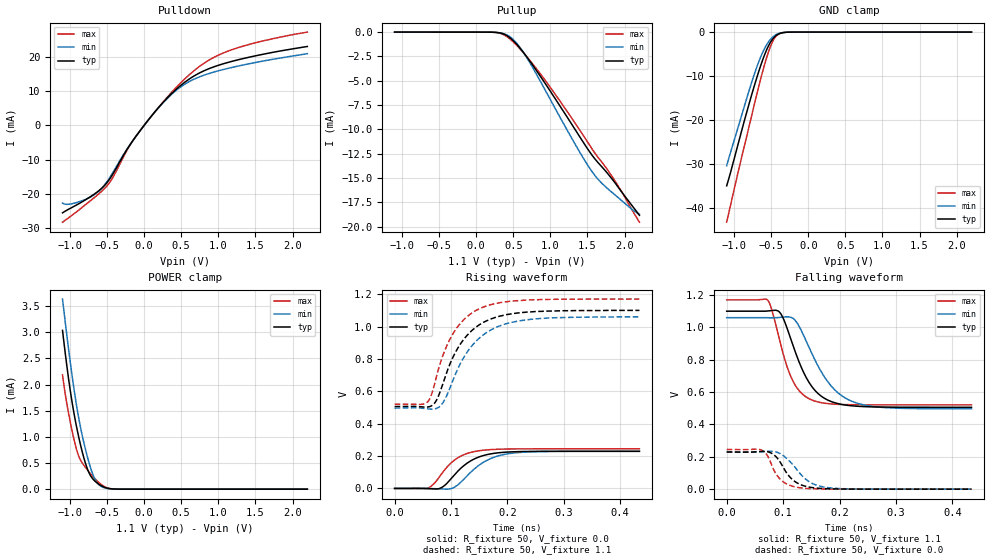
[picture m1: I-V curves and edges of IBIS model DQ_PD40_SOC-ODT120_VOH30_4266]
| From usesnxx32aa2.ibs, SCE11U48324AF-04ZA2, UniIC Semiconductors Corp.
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| DQ_PD40_SOC-ODT120_VOH30_4266
| (40 Ohm Pulldown, 120 Ohm System ODT Setting, VOH=VDDQ/3.0, 3200-4266Mbps)
[Model]   DQ_PD40_SOC-ODT120_VOH30_4266
Model_type   I/O
Vinl = 123.333mV
Vinh = 243.333mV
Vmeas = 183.333mV
Vref = 0.0mV
Cref = 0.0pF
Rref = 120.000Ohm
|   typ   min   max
|C_comp   0.797pF   0.747pF   0.847pF
C_comp_pullup   0.3985pF   0.3735pF   0.4235pF
C_comp_pulldown   0.3985pF   0.3735pF   0.4235pF
| Note: C_comp changes when the ODT circuit is enabled.
[Model Spec]
| Input threshold voltage corners
Vinl   0.1233V   0.1167V   0.1350V
Vinh   0.2433V   0.2367V   0.2550V
| Measurement voltage corners
Vmeas   0.1833V   0.1767V   0.1950V
| Timing spec test load voltage corners
Vref   0.0000V   0.0000V   0.0000V
| Dynamic Overshoot Parameters from LPDDR4 Specification
D_overshoot_ampl_h   0.30   NA   NA
D_overshoot_ampl_l   0.30   NA   NA
D_overshoot_area_h   0.1n   NA   NA
D_overshoot_area_l   0.1n   NA   NA
[Receiver Thresholds]
Vth   = 0.1833V
Vth_min  = 0.1800V
Vth_max  = 0.1866V
Vinh_ac  = 0.060V
Vinh_dc  = 0.060V
Vinl_ac  = -0.060V
Vinl_dc  = -0.060V
Tslew_ac = 5.000ns |Not specified, so set to high value
Threshold_sensitivity = 0.1667
Reference_supply Pullup_ref
[Voltage Range]   1.1000V   1.0600V   1.1700V
[Pullup Reference]   1.1000V   1.0600V   1.1700V
| Junction Temperature (Ambient temp is 35C typ 95C min -40C max)
[Temperature Range]   50.0   110.0   -40.0
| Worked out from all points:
|   slope of the pulldown table from 0 to 0.165 V, typ, clamps not added: 37 ohm
|   slope of the pullup table from 0 to 0.165 V, typ, clamps not added: 39.2 kohm
|   GND clamp passes 1 mA (typ) near -0.45 V on its own axis
|   POWER clamp passes 1 mA (typ) near -0.88 V on its own axis
|   rising waveform, R_fixture 50, V_fixture 0.0: 20-80 % time 45.7ps typ, 49.8ps min, 40.7ps max; typ from 0 V to 0.23 V
|   falling waveform, R_fixture 50, V_fixture 1.1: 20-80 % time 44.6ps typ, 56.1ps min, 34.9ps max; typ from 1.1 V to 0.506 V
|   rising waveform, R_fixture 50, V_fixture 1.1: 20-80 % time 55.4ps typ, 59.8ps min, 50.8ps max; typ from 0.506 V to 1.1 V
|   falling waveform, R_fixture 50, V_fixture 0.0: 20-80 % time 29.8ps typ, 37.9ps min, 24.9ps max; typ from 0.23 V to 0 V
[Pulldown]
|   Voltage   I(typ)   I(min)   I(max)
-1.1V     -25.52mA   -22.67mA   -28.25mA
-1.018V   -24.47mA   -23.02mA   -26.96mA
-869mV    -22.73mA   -22.24mA   -24.52mA
-614.9mV  -19.15mA   -19.26mA   -20.05mA
-459.8mV  -15.51mA   -15.11mA   -16.51mA
-159.5mV  -4.698mA   -4.697mA   -4.713mA
163.9mV   4.425mA    4.387mA    4.447mA
457.6mV   11mA       10.65mA    11.62mA
721.6mV   15mA       13.93mA    16.78mA
942.7mV   17.09mA    15.56mA    19.86mA
1.233V    18.95mA    17.13mA    22.43mA
2.2V      23.01mA    20.92mA    27.21mA
[GND Clamp]
|   Voltage   I(typ)   I(min)   I(max)
-1.1V     -34.88mA   -30.34mA   -43.13mA
-1.047V   -31.79mA   -27.25mA   -39.23mA
-938.3mV  -24.92mA   -21.15mA   -31.24mA
-789.8mV  -15.79mA   -12.83mA   -20.82mA
-664.4mV  -8.768mA   -6.598mA   -12.12mA
-595.1mV  -5.416mA   -3.908mA   -7.721mA
-522.5mV  -2.672mA   -1.905mA   -3.823mA
-469.7mV  -1.358mA   -986.2uA   -1.793mA
-413.6mV  -565.2uA   -417.3uA   -622.1uA
-350.9mV  -166.3uA   -125.9uA   -147.8uA
-228.8mV  -6.714uA   -6.472uA   -3.562uA
2.2V      0A         0A         0A
[Pullup]
|   Voltage   I(typ)   I(min)   I(max)
-1.1V     2.095uA    3.229uA    944.5nA
233.2mV   -16.16uA   -16.42uA   -16.87uA
342.1mV   -127.3uA   -105.3uA   -175.8uA
437.8mV   -483.6uA   -396.2uA   -609uA
556.6mV   -1.343mA   -1.244mA   -1.449mA
685.3mV   -2.586mA   -2.666mA   -2.557mA
952.6mV   -5.54mA    -6.28mA    -5.194mA
1.319V    -9.846mA   -11.33mA   -9.205mA
1.586V    -12.9mA    -14.6mA    -12.28mA
1.692V    -13.83mA   -15.53mA   -13.35mA
1.867V    -15.45mA   -16.71mA   -15.25mA
2.2V      -18.83mA   -18.71mA   -19.54mA
[POWER Clamp]
|   Voltage   I(typ)   I(min)   I(max)
-1.1V     3.036mA    3.636mA    2.186mA
-1.044V   2.383mA    2.969mA    1.653mA
-977.9mV  1.724mA    2.242mA    1.161mA
-908.6mV  1.178mA    1.582mA    748.6uA
-852.5mV  818.7uA    1.149mA    543.7uA
-779.9mV  448.2uA    701.9uA    396.3uA
-713.9mV  239.3uA    373.1uA    278.6uA
-661.1mV  151.1uA    187.6uA    195.5uA
-598.4mV  83.65uA    71.97uA    113.1uA
-489.5mV  17.8uA     10.83uA    22.45uA
-377.3mV  1.498uA    1.063uA    1.232uA
2.2V      0A         0A         0A
[Ramp]
|   typ   min   max
| 20% - 80%
dV/dt_r   137.88m/45.74p   137.44m/49.83p   147.06m/40.67p
dV/dt_f   356.26m/44.55p   338.01m/56.12p   389.46m/34.89p
| 25% - 75%
|dV/dt_r   114.90m/36.50p   114.53m/39.79p   122.55m/32.29p
|dV/dt_f   296.88m/35.55p   281.68m/44.83p   324.55m/27.77p
R_load = 50
[Rising Waveform]
R_fixture = 50
V_fixture = 0.0
|   Time   V(typ)   V(min)   V(max)
0s        163.8uV    121.7uV    125.4uV
58ps      -597.2uV   381.8uV    1.108mV
69ps      -2.733mV   -889.7uV   27.23mV
80ps      703.6uV    -2.773mV   74.58mV
107ps     88.01mV    9.696mV    177.6mV
126ps     150mV      69.17mV    213.2mV
146ps     189.8mV    134.1mV    231.2mV
176ps     217mV      192.7mV    241.2mV
217ps     227.5mV    221.3mV    244.5mV
434ps     230mV      229.2mV    245.2mV
[Falling Waveform]
R_fixture   = 50
V_fixture   = 1.1
V_fixture_min = 1.06
V_fixture_max = 1.17
|   Time   V(typ)   V(min)   V(max)
0s        1.1V       1.06V      1.17V
73ps      1.101V     1.06V      1.167V
79ps      1.104V     1.059V     1.12V
95ps      1.089V     1.062V     903.8mV
114ps     924.7mV    1.062V     693.9mV
125ps     816.3mV    1.027V     624.2mV
149ps     643.9mV    853.4mV    554.1mV
185ps     542mV      638.7mV    526.9mV
226ps     513.9mV    537.6mV    521.8mV
434ps     506.2mV    496.6mV    520.9mV
[Rising Waveform]
R_fixture   = 50
V_fixture   = 1.1
V_fixture_min = 1.06
V_fixture_max = 1.17
|   Time   V(typ)   V(min)   V(max)
0s        506.1mV    496.4mV    520.9mV
58ps      502.9mV    491.9mV    533.3mV
66ps      511.7mV    489.9mV    585.9mV
80ps      590.9mV    506.7mV    763.3mV
95ps      742.2mV    594.4mV    900.4mV
113ps     872.5mV    746.2mV    1.005V
133ps     962.6mV    863.7mV    1.074V
156ps     1.023V     945.8mV    1.119V
236ps     1.09V      1.043V     1.164V
434ps     1.1V       1.06V      1.17V
[Falling Waveform]
R_fixture = 50
V_fixture = 0.0
|   Time   V(typ)   V(min)   V(max)
0s        230mV      229.3mV    245.3mV
60ps      233mV      230.4mV    243.7mV
70ps      232.6mV    233.3mV    218mV
78ps      224.9mV    234.3mV    163.6mV
97ps      154.6mV    215.3mV    54.68mV
111ps     79.09mV    174.9mV    24.95mV
127ps     34.46mV    109.7mV    10.38mV
151ps     10.15mV    36.8mV     2.938mV
185ps     2.09mV     7.415mV    619.5uV
434ps     237.1uV    226uV      152.9uV
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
